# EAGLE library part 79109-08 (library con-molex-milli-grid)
RECEPTACAL
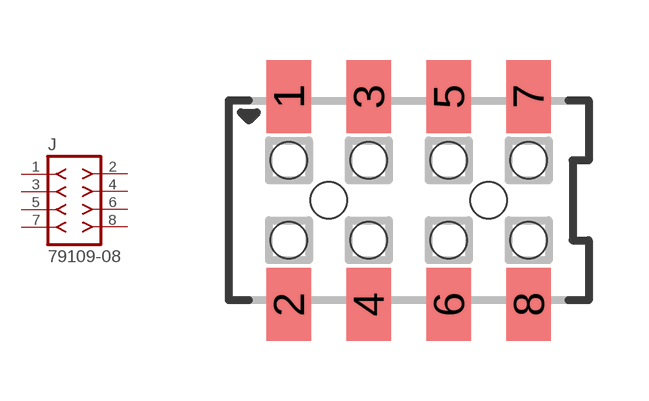
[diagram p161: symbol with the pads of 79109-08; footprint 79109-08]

Designator prefix J

## 79109-08  [79109-08]
1  1  pas
2  2  pas
3  3  pas
4  4  pas
5  5  pas
6  6  pas
7  7  pas
8  8  pas

## Footprint 79109-08 (pad centres in mm)
RECEPTACAL SMD Dual Row, Vertical, Pass-Thru
smd 1.12 x 1.83: 1 -3,2.6; 2 -3,-2.6; 3 -1,2.6; 4 -1,-2.6; 5 1,2.6; 6 1,-2.6; 7 3,2.6; 8 3,-2.6
hole 0.914 at -2,0
hole 0.914 at -3,1
hole 0.914 at -3,-1
hole 0.914 at -1,-1
hole 0.914 at -1,1
hole 0.914 at 1,-1
hole 0.914 at 1,1
hole 0.914 at 2,0
hole 0.914 at 3,1
hole 0.914 at 3,-1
